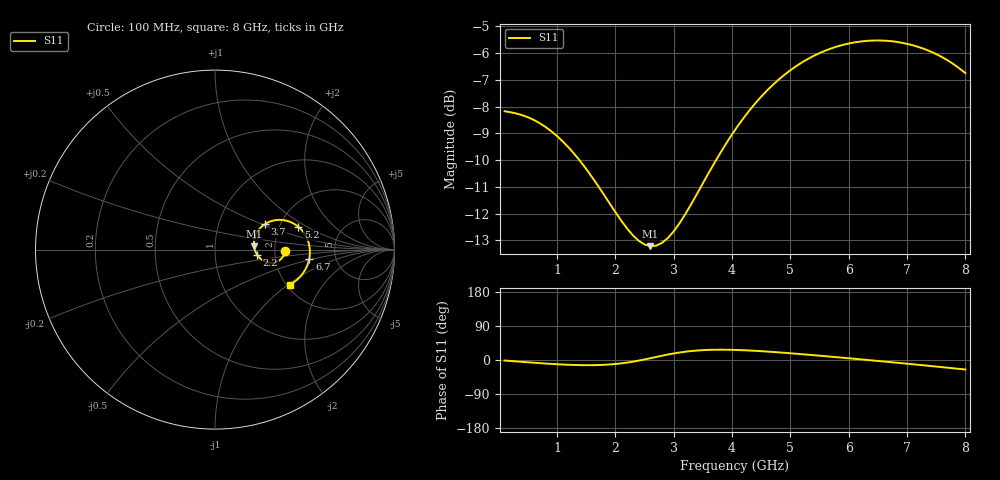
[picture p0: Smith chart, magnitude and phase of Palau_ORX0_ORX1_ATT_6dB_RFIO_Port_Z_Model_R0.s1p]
! Created Fri Jul 10 10:45:06 2020
! Palau ORX0/ORX1 RFIO Port Impedance Model.
! Attenuation : 6 dB.
! Revision		: R0.
! Impedance Mode 	: Balanced Differential-Mode.
! Impedance Format 	: Series Equivalent Differential Impedance (SEDZ).
# hz S ma R 50
! 1 Port Network Data from SP1.SP block
! freq  magS11  angS11
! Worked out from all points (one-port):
!   80 points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, 100 MHz to 8 GHz, reference 50 ohm
!   lowest |S11| = -13.2 dB at 2.6 GHz (marker M1), VSWR 1.56, Z = 77.8 + j2.94 ohm
!   |S11| at or under -10 dB: 1.382 GHz to 3.725 GHz (2.343 GHz wide, 91.7 % of centre)
!   S11 on the Smith chart (normalised r, x): 100 MHz: 2.28, -0.05; 2.2 GHz: 1.61, -0.10; 3.7 GHz: 1.67, +0.53; 5.2 GHz: 2.54, +0.84; 6.7 GHz: 3.17, -0.44; 8 GHz: 2.08, -1.03
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1e8  0.3903 -1.4
6e8  0.376 -7.2
9e8  0.3581 -10.3
1.1e9  0.3425 -12.0
1.4e9  0.3145 -13.5
1.6e9  0.2939 -13.6
1.8e9  0.2729 -12.7
2.1e9  0.2438 -8.9
2.2e9  0.2357 -6.8
2.4e9  0.2236 -1.6
2.6e9  0.2185 4.7
2.8e9  0.2216 11.3
2.9e9  0.2263 14.5
3.1e9  0.2412 19.8
3.4e9  0.2737 25.0
3.7e9  0.3129 27.1
4.1e9  0.3666 26.3
4.3e9  0.3919 25.0
4.6e9  0.4267 22.3
5.1e9  0.4739 16.5
5.2e9  0.4816 15.3
5.7e9  0.5113 8.7
6.1e9  0.5247 3.2
6.4e9  0.5289 -1.1
6.7e9  0.5279 -5.4
7.1e9  0.5182 -11.3
7.5e9  0.4989 -17.3
8e9  0.4599 -25.1
